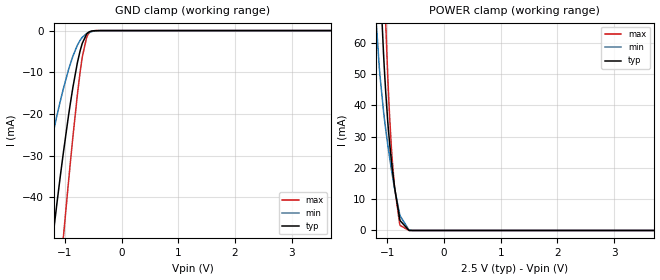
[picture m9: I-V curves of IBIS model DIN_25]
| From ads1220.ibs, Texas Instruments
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|   DIN_25 Model
[Model]   DIN_25
Model_type   Input
Vinl = .69
Vinh = 1.89
|   typ   min   max
|   (nom PVT)   (Fast PVT)   (slow PVT)
C_comp   6.893p   6.429p   7.322p
| Where   nom PVT is  Nominal Process, 2.5V, 27C
|   Fast PVT is Strong Process, 2.7V, -40C
|   Slow PVT is Weak Process, 2.3V, 125C
[Voltage Range]   2.5   2.3   2.7
[Temperature Range]   27   125   -40
[Power Clamp Reference]   2.5   2.3   2.7
[GND Clamp Reference]   0   0   0
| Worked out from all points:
|   GND clamp passes 1 mA (typ) near -0.62 V on its own axis
|   POWER clamp passes 1 mA (typ) near -0.67 V on its own axis
[GND Clamp]
|   Voltage   I(typ)   I(min)   I(max)
-2.5V     -222.2mA   -135.1mA   -291.4mA
-1.615V   -99.96mA   -54.22mA   -144.3mA
-1.488V   -83.4mA    -44.23mA   -123.2mA
-1.225V   -51.16mA   -25.71mA   -80.54mA
-1.143V   -41.75mA   -20.56mA   -67.49mA
-1.03V    -29.69mA   -14.15mA   -50.18mA
-865mV    -14.2mA    -6.414mA   -26.44mA
-730mV    -4.813mA   -2.307mA   -9.867mA
-692.5mV  -3.053mA   -1.611mA   -6.302mA
-617.5mV  -885.9uA   -722.2uA   -1.735mA
-565mV    -282.9uA   -386.4uA   -493.8uA
5V        0A         0A         0A
[POWER Clamp]
|   Voltage   I(typ)   I(min)   I(max)
-2.5V     812.1mA    603.1mA    1.021A
-1.24V    131mA      78.22mA    188.3mA
-1.143V   86.15mA    52.21mA    129mA
-1.127V   79.78mA    49mA       120.2mA
-1.067V   56.56mA    38.09mA    86.34mA
-1.03V    44.51mA    32.47mA    66.76mA
-962.5mV  28.32mA    23.63mA    37.17mA
-917.5mV  20.44mA    18.3mA     23.36mA
-872.5mV  13.78mA    13.36mA    13.78mA
-775mV    3.144mA    4.66mA     1.621mA
-617.5mV  15.03uA    137.5uA    1.062uA
5V        0A         0A         0A
